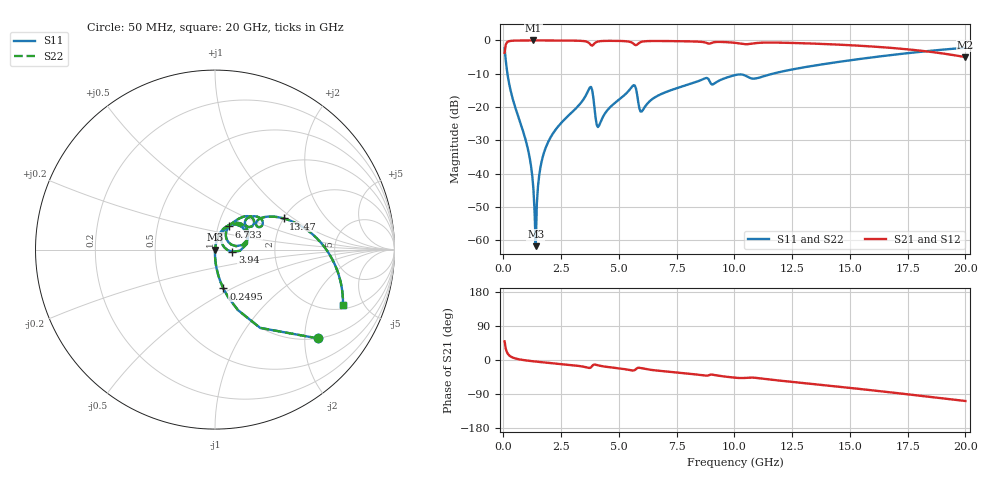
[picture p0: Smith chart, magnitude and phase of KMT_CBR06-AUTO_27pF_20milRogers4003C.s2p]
! Data measured by Modelithics Inc. support@modelithics.com 813-866-6335
! KEMET CBR06-AUTO 27pF, Pad Width= 0.851mm, Pad Length= 0.64mm, Pad Gap= 0.62mm, 20mil Rogers 4003C substrate Data, January 2022
# hz S ma R 50
! 2 Port Network Data from SP1.SP block
! freq  magS11  angS11  magS21  angS21  magS12  angS12  magS22  angS22
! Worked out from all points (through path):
!   401 points, 50 MHz to 20 GHz, reference 50 ohm
!   highest |S21| = -0.01 dB at 1.297 GHz (marker M1); lowest = -5.0 dB at 20 GHz (marker M2)
!   group delay of S21, straight-line fit = 15.2 ps
!   lowest |S11| = -61.8 dB at 1.397 GHz (marker M3), VSWR 1.00, Z = 50.1 + j0.0434 ohm
!   |S11| at or under -10 dB: 174.1 MHz to 11.65 GHz (11.48 GHz wide, 194 % of centre)
!   |S22| runs from -61.8 to -2.2 dB; largest |S21 - S12| = 0
!   S11 on the Smith chart (normalised r, x): 50 MHz: 0.99, -2.33; 249.5 MHz: 0.99, -0.45; 3.94 GHz: 1.21, -0.03; 6.733 GHz: 1.13, +0.30; 13.47 GHz: 2.00, +0.84; 20 GHz: 2.23, -3.48
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5e7  0.7597 -40.7  0.65 49.3  0.65 49.3  0.7597 -40.7
2.495e8  0.2214 -77.9  0.9748 12.1  0.9748 12.1  0.2214 -77.9
1.0475e9  0.02438 -90.4  0.9991 -1.7  0.9991 -1.7  0.02438 -90.4
1.197125e9  0.01278 -90.1  0.9993 -2.8  0.9993 -2.8  0.01278 -90.1
1.296875e9  0.005924 -87.4  0.9993 -3.5  0.9993 -3.5  0.005924 -87.4
1.396625e9  0.0008173 32.0  0.9993 -4.1  0.9993 -4.1  0.0008173 32.0
1.496375e9  0.006498 79.1  0.9992 -4.8  0.9992 -4.8  0.006498 79.1
1.54625e9  0.009357 80.6  0.9992 -5.1  0.9992 -5.1  0.009357 80.6
1.646e9  0.01489 81.5  0.9991 -5.7  0.9991 -5.7  0.01489 81.5
1.895375e9  0.0279 81.1  0.9987 -7.2  0.9987 -7.2  0.0279 81.1
3.391625e9  0.1202 69.0  0.984 -16.9  0.984 -16.9  0.1202 69.0
3.74075e9  0.1968 40.2  0.8899 -20.9  0.8899 -20.9  0.1968 40.2
3.94025e9  0.09763 -7.3  0.9025 -12.1  0.9025 -12.1  0.09763 -7.3
4.13975e9  0.05281 43.1  0.9707 -14.7  0.9707 -14.7  0.05281 43.1
5.586125e9  0.206 44.4  0.9172 -27.7  0.9172 -27.7  0.206 44.4
5.985125e9  0.08578 38.8  0.955 -21.9  0.955 -21.9  0.08578 38.8
6.73325e9  0.1512 58.7  0.9808 -28.4  0.9808 -28.4  0.1512 58.7
1.0025e10  0.3016 37.0  0.9204 -46.7  0.9204 -46.7  0.3016 37.0
1.336662e10  0.4141 25.1  0.8977 -63.2  0.8977 -63.2  0.4141 25.1
1.346638e10  0.4195 24.5  0.8951 -63.9  0.8951 -63.9  0.4195 24.5
1.670825e10  0.5991 2.7  0.7767 -85.0  0.7767 -85.0  0.5991 2.7
2e10  0.7769 -23.4  0.5616 -108.2  0.5616 -108.2  0.7769 -23.4
